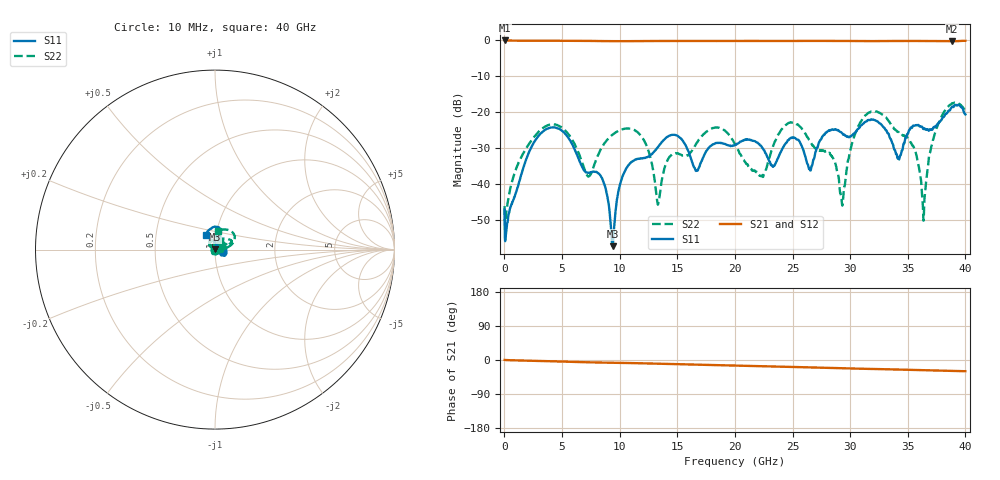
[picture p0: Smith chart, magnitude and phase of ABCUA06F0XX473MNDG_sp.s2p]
! Amotech Co.,Ltd.
! http://www.amotech.co.kr/
! Date: Wednesday, December 02, 2020 16:36:14
! Part Number: ABCUA 06F 0XX 473M NDG
! Freq. Start=10[MHz] Stop=40[GHz], 4000[Steps]
# Hz S  dB  R 50
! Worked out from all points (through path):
!   4000 points, 10 MHz to 40 GHz, reference 50 ohm
!   highest |S21| = 0.00 dB at 30 MHz (marker M1); lowest = -0.2 dB at 38.8 GHz (marker M2)
!   group delay of S21, straight-line fit = 2.03 ps
!   lowest |S11| = -57.2 dB at 9.38 GHz (marker M3), VSWR 1.00, Z = 50.1 + j0.0729 ohm
!   |S11| at or under -10 dB: start of sweep to end of sweep
!   |S22| runs from -51.3 to -17.2 dB; largest |S21 - S12| = 0.0035
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1e7  -47.05 -110.8  -0.01 0.2  0.00 0.3  -46.04 -57.2
3e7  -54.38 -153.1  -0.00 0.0  0.00 0.0  -50.86 -18.0
3.41e9  -25.11 125.7  -0.08 -2.8  -0.07 -2.7  -24.16 43.4
6.68e9  -34.71 56.6  -0.10 -5.6  -0.09 -5.6  -33.39 59.0
8.48e9  -38.43 -33.6  -0.18 -6.8  -0.17 -6.8  -29.59 -21.7
9.38e9  -57.18 31.7  -0.20 -7.3  -0.19 -7.2  -26.17 -9.7
1.047e10  -36.23 99.6  -0.21 -7.8  -0.19 -7.8  -24.53 11.2
1.222e10  -32.64 41.4  -0.17 -8.9  -0.16 -8.9  -28.50 40.1
1.334e10  -29.53 -15.5  -0.16 -9.7  -0.14 -9.7  -45.43 138.9
1.452e10  -26.26 -40.2  -0.15 -10.6  -0.14 -10.5  -31.74 -127.5
1.666e10  -36.19 25.6  -0.15 -12.2  -0.14 -12.1  -28.55 -9.6
2.001e10  -29.06 23.8  -0.14 -14.7  -0.13 -14.6  -28.78 77.8
2.228e10  -29.36 -21.4  -0.14 -16.3  -0.12 -16.2  -37.66 -107.7
2.453e10  -28.09 91.3  -0.15 -18.0  -0.13 -17.9  -23.21 11.7
2.667e10  -34.86 16.8  -0.13 -19.6  -0.12 -19.6  -28.84 64.1
2.929e10  -25.71 3.1  -0.14 -21.7  -0.13 -21.6  -45.43 103.7
3.097e10  -23.59 79.3  -0.17 -23.0  -0.15 -22.9  -22.33 20.0
3.334e10  -25.98 70.8  -0.16 -24.6  -0.14 -24.5  -22.41 53.9
3.554e10  -23.68 -27.2  -0.15 -26.2  -0.14 -26.1  -29.86 147.1
3.638e10  -24.58 2.0  -0.16 -26.9  -0.14 -26.8  -50.02 68.0
3.88e10  -18.63 75.4  -0.25 -28.9  -0.23 -28.8  -17.59 33.1
4e10  -20.55 124.2  -0.10 -29.5  -0.08 -29.4  -19.68 82.3
